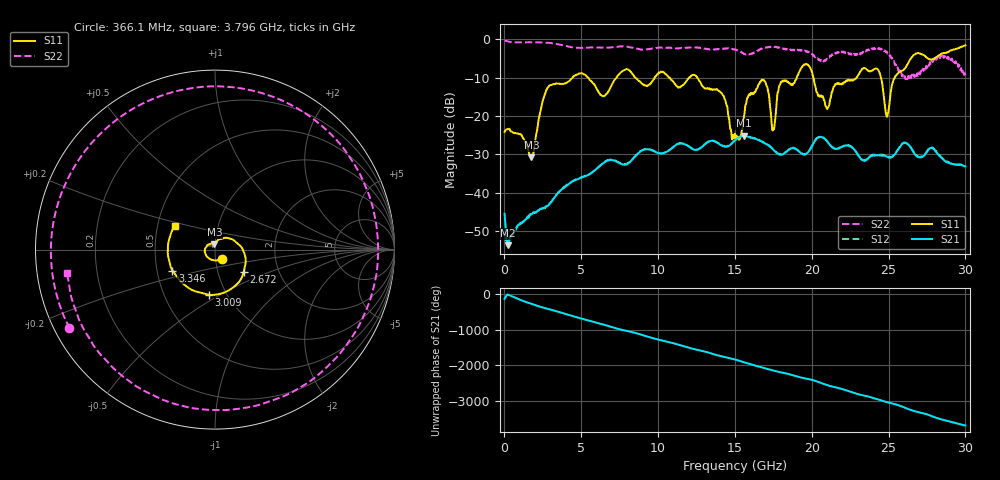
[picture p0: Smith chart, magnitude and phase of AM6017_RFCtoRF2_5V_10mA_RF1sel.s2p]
!Agilent Technologies,E8364B,MY43040894,A.07.50.67
!Agilent E8364B: A.07.50.67
!Date: Tuesday, August 21, 2018 13:39:02
!Correction: S11(Full 2 Port(1,2))
!S21(Full 2 Port(1,2))
!S12(Full 2 Port(1,2))
!S22(Full 2 Port(1,2))
!S2P File: Measurements: S11, S21, S12, S22:
# Hz S  dB  R 50
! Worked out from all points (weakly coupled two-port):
!   1601 points, 10 MHz to 30 GHz, reference 50 ohm
!   highest |S21| = -25.13 dB at 15.59 GHz (marker M1); lowest = -53.6 dB at 216.2 MHz (marker M2)
!   lowest |S11| = -30.7 dB at 1.753 GHz (marker M3), VSWR 1.06, Z = 49.6 + j2.86 ohm
!   |S11| at or under -10 dB: start of sweep to 4.433 GHz; 12.55 GHz to 19.02 GHz (6.476 GHz wide, 41 % of centre); 20.11 GHz to 22.92 GHz (2.815 GHz wide, 13.1 % of centre)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
!   |S22| runs from -10.4 to -0.3 dB; largest |S21 - S12| = 0.0082
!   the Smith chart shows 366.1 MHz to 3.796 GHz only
!   S11 on the Smith chart (normalised r, x): 366.1 MHz: 1.08, -0.11; 2.672 GHz: 1.33, -0.34; 3.009 GHz: 0.83, -0.44; 3.346 GHz: 0.60, -0.15; 3.796 GHz: 0.61, +0.17
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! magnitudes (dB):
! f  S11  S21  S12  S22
! 10 MHz  -24.1  -45.5  -50.8  -0.3
! 216.2 MHz  -23.4  -53.6  -53.7  -0.6
! 366.1 MHz  -23.7  -51.5  -52.2  -0.7
! 1.753 GHz  -30.7  -45.6  -45.4  -0.8
! 2.672 GHz  -13.9  -43.7  -43.8  -0.9
! 3.009 GHz  -11.9  -42.6  -42.5  -1.0
! 3.346 GHz  -11.6  -40.7  -40.7  -1.2
! 3.796 GHz  -11.7  -38.9  -38.8  -1.6
! 5.015 GHz  -8.8  -36.0  -36.0  -2.3
! 10.02 GHz  -8.9  -29.7  -29.5  -2.3
! 13.97 GHz  -13.6  -27.3  -27.2  -2.6
! 15.01 GHz  -24.6  -26.4  -26.3  -2.8
! 15.59 GHz  -20.1  -25.1  -25.0  -3.9
! 16.84 GHz  -10.6  -26.9  -26.8  -2.3
! 17.5 GHz  -23.6  -28.8  -28.6  -2.0
! 18.02 GHz  -11.2  -30.1  -29.9  -2.3
! 20.01 GHz  -8.5  -27.9  -27.8  -3.8
! 21 GHz  -18.2  -26.6  -26.5  -5.2
! 24.21 GHz  -7.6  -30.2  -30.1  -2.5
! 25.01 GHz  -18.1  -30.9  -30.7  -3.8
! 26.68 GHz  -4.0  -29.7  -29.6  -9.8
! 30 GHz  -1.6  -33.1  -32.9  -9.3
